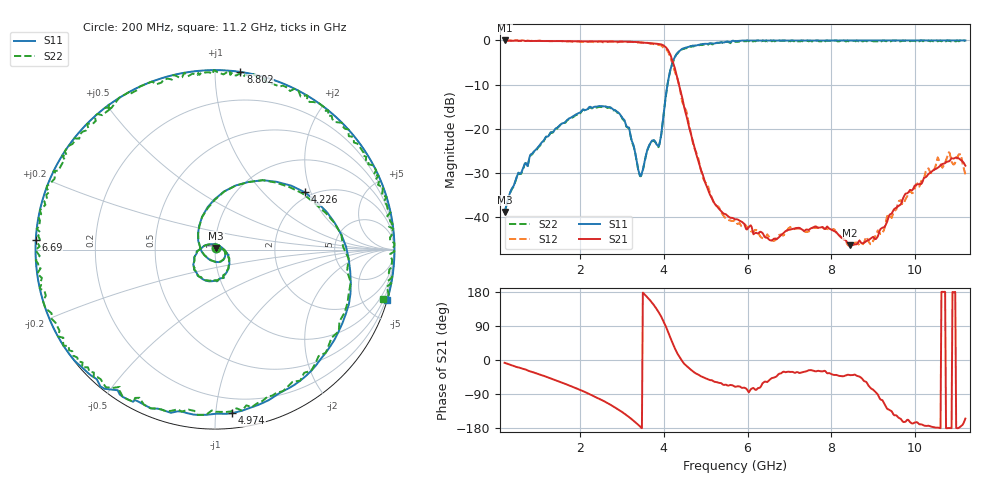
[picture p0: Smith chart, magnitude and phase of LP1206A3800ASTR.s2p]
!	AVX	THIN	FILM	OPERATION
!	LP1206	High	Performance	Low	Pass	Filters
!	P/N	LP1206A3800ASTR	18	October	2017
!Instrument:	"HEWLETT PACKARD,8720ES,US39172150,7.62 "
#	MHz	S	dB	R	50
!	Frq	S11(dB)	S11(deg)	S21(dB)	S21(deg)	S12(dB)	S12(deg)	S22(dB)	S22(deg)
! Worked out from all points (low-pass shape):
!   501 points, 200 MHz to 11.2 GHz, reference 50 ohm
!   highest |S21| = 0.00 dB at 200 MHz (marker M1); lowest = -46.4 dB at 8.45 GHz (marker M2)
!   |S21| within 3 dB of the highest: start of sweep to 4.145 GHz
!   lowest |S11| = -38.9 dB at 200 MHz (marker M3), VSWR 1.02, Z = 50.7 + j0.893 ohm
!   |S11| at or under -10 dB: start of sweep to 4.089 GHz
!   |S22| runs from -39.1 to 0.0 dB; largest |S21 - S12| = 0.052
!   S11 on the Smith chart (normalised r, x): 200 MHz: 1.01, +0.02; 4.226 GHz: 1.84, +1.82; 4.974 GHz: 0.10, -1.10; 6.69 GHz: 0.00, +0.03; 8.802 GHz: 0.00, +1.15; 11.2 GHz: 0.00, -6.97
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200  -38.89 50.8  0.00 -7.4  -0.03 -7.2  -39.09 50.7
860  -25.64 -0.9  -0.13 -31.6  -0.07 -31.8  -25.84 -1.1
2048  -15.90 -72.7  -0.20 -81.1  -0.31 -81.4  -15.90 -72.8
2906  -16.31 -140.3  -0.21 -130.1  -0.38 -129.2  -16.31 -140.5
3324  -25.79 148.2  -0.34 -164.6  -0.44 -164.2  -25.89 148.1
3456  -30.68 65.4  -0.47 -177.8  -0.47 -177.7  -30.78 65.4
3676  -23.34 -35.1  -0.62 157.1  -0.72 156.5  -23.34 -35.2
3874  -24.00 -132.3  -0.80 126.7  -1.00 125.9  -24.20 -132.5
4050  -12.40 99.9  -1.55 88.3  -1.91 89.6  -12.60 99.9
4226  -4.53 32.5  -5.13 40.5  -5.90 41.6  -4.73 32.5
4446  -1.88 -22.1  -13.22 -3.9  -14.04 0.6  -1.98 -22.1
4688  -1.20 -56.8  -22.64 -29.4  -22.93 -30.6  -1.20 -56.9
4974  -0.76 -84.1  -31.81 -47.4  -31.96 -44.5  -0.86 -84.3
5700  -0.20 -132.4  -40.55 -70.7  -40.74 -71.8  -0.30 -132.6
6690  0.00 176.9  -45.12 -43.5  -44.75 -37.0  -0.20 176.7
7548  0.00 136.4  -42.47 -27.5  -42.54 -26.1  -0.20 136.2
8450  0.00 96.0  -46.41 -40.0  -46.65 -39.5  -0.20 95.8
8802  0.00 81.9  -45.73 -56.4  -45.25 -54.5  -0.10 81.9
9374  0.00 59.1  -39.83 -131.0  -39.55 -132.1  0.00 59.0
10540  0.00 11.1  -28.89 -178.4  -26.52 -177.8  -0.20 11.0
11068  0.00 -10.6  -26.94 -177.1  -25.82 177.2  0.00 -10.8
11200  0.00 -16.3  -28.40 -154.6  -30.34 -160.4  -0.20 -16.3
